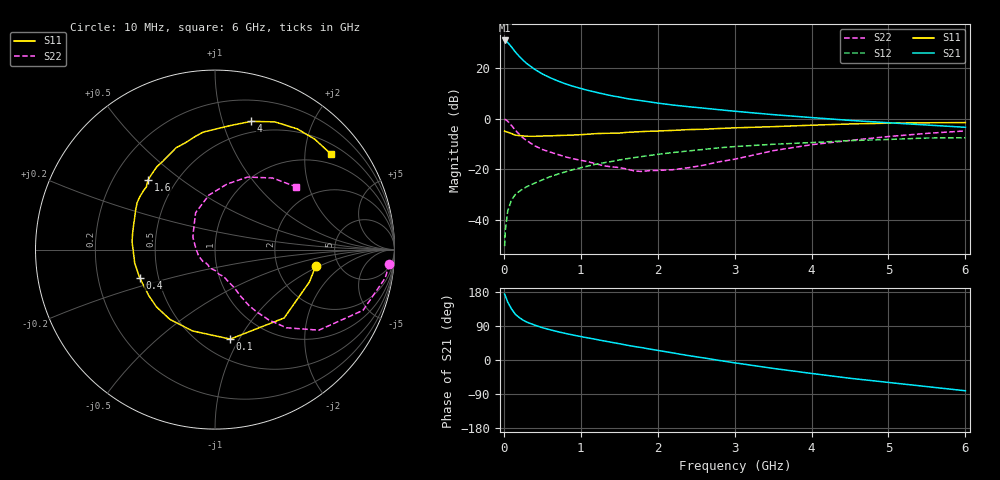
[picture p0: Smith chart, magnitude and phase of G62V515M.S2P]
! SIEMENS Small Signal Semiconductors
! BFG193
! Si NPN RF Bipolar Junction Transistor in SOT223
! VCE = 2.5 V  IC = 15 mA
! Common Emitter S-Parameters:  August  1996
# GHz  S  MA  R  50
!  f  S11  S21  S12  S22
! GHz  MAG  ANG  MAG  ANG  MAG  ANG  MAG  ANG
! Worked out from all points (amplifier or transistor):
!   36 points, 10 MHz to 6 GHz, reference 50 ohm
!   highest |S21| = 30.9 dB at 10 MHz (marker M1)
!   |S21| within 3 dB of that: start of sweep to 110.5 MHz
!   unconditionally stable (mu >= 1): 747.8 MHz to 2.63 GHz
!   at 250 MHz: K = 0.66, MSG = 25.4 dB, |S12| = -27.8 dB
!   at 1.4 GHz: K = 1.06, MAG = 11.5 dB, |S12| = -16.9 dB
!   at 6 GHz: K = 0.90, MSG = 2.1 dB, |S12| = -7.5 dB
!   S11 on the Smith chart (normalised r, x): 10 MHz: 3.35, -0.93; 100 MHz: 0.69, -0.92; 400 MHz: 0.39, -0.15; 1.6 GHz: 0.35, +0.38; 4 GHz: 0.39, +1.25; 6 GHz: 0.73, +2.60
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0.01  0.5681 -9.5  35.27 174.0  0.003 88.6  0.975 -4.7
0.02  0.5561 -18.9  34.89 169.1  0.0062 83.1  0.9613 -9.5
0.05  0.5418 -44.7  32.18 153.0  0.0148 72.2  0.8915 -22.3
0.1  0.5057 -80.3  26.2 134.7  0.0249 62.9  0.7325 -37.8
0.15  0.4702 -105.4  20.83 120.6  0.0316 56.3  0.5897 -47.6
0.2  0.463 -122.8  17.13 112.1  0.0364 55.2  0.4929 -52.6
0.25  0.4563 -135.6  14.32 105.2  0.0409 54.1  0.4156 -56.3
0.3  0.4492 -145.3  12.26 99.9  0.0452 54.9  0.3657 -58.7
0.4  0.4481 -159.6  9.497 92.2  0.053 55.2  0.2914 -61.4
0.5  0.4538 -170.5  7.672 85.3  0.0614 55.6  0.246 -62.8
0.6  0.4554 -178.9  6.476 79.9  0.0708 56.0  0.2188 -64.7
0.7  0.4642 174.6  5.585 74.8  0.0797 56.1  0.1961 -67.2
0.9  0.4739 163.0  4.373 65.9  0.0983 54.2  0.1607 -71.5
1.1  0.4938 153.6  3.606 58.1  0.116 52.3  0.14 -80.4
1.6  0.537 134.1  2.5 39.1  0.1615 44.1  0.1007 -109.4
2.2  0.586 115.9  1.861 18.6  0.2138 32.0  0.0979 -162.6
2.8  0.6395 100.0  1.503 -1.1  0.265 19.0  0.1405 151.3
3.5  0.6944 83.4  1.202 -22.1  0.3112 2.4  0.2323 117.7
4  0.7426 74.2  1.051 -35.5  0.3367 -7.2  0.3054 96.4
4.5  0.7858 64.9  0.924 -48.2  0.3678 -17.4  0.3714 79.6
5.5  0.829 47.9  0.749 -70.2  0.4144 -40.8  0.5118 51.2
6  0.8369 39.6  0.675 -81.2  0.4196 -54.3  0.5725 37.6
